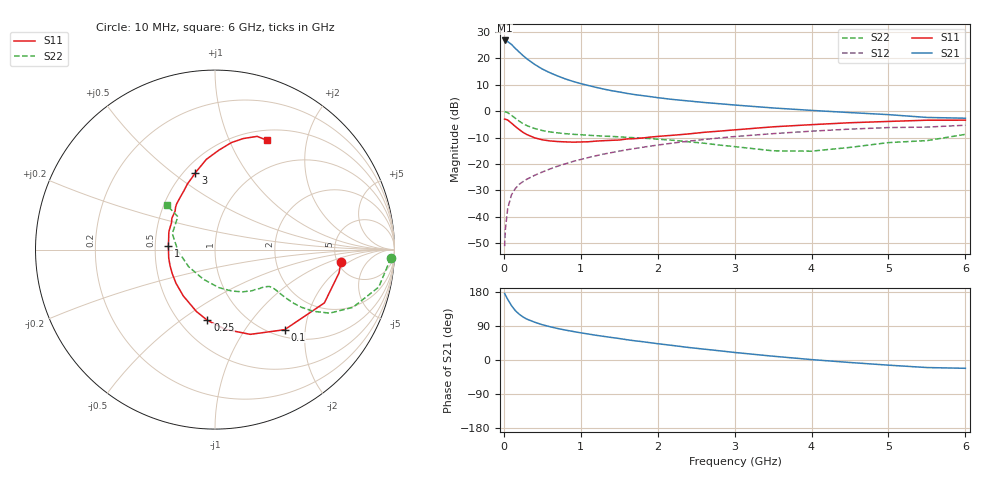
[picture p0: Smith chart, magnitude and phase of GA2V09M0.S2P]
! Infineon Technologies  Discrete & RF Semiconductors
! BF775
! Si NPN RF Bipolar Junction Transistor in SOT23
! VCE = 2 V  IC = 9 mA
! Common Emitter S-Parameters:  May  1996
# GHz  S  MA  R  50
!  f  S11  S21  S12  S22
! GHz  MAG  ANG  MAG  ANG  MAG  ANG  MAG  ANG
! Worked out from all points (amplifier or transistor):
!   36 points, 10 MHz to 6 GHz, reference 50 ohm
!   highest |S21| = 26.7 dB at 10 MHz (marker M1)
!   |S21| within 3 dB of that: start of sweep to 149.3 MHz
!   unconditionally stable (mu >= 1): 562.9 MHz to 3.79 GHz
!   at 250 MHz: K = 0.67, MSG = 23.8 dB, |S12| = -26.6 dB
!   at 1.4 GHz: K = 1.13, MAG = 9.5 dB, |S12| = -15.7 dB
!   at 6 GHz: K = 0.98, MSG = 1.3 dB, |S12| = -5.3 dB
!   S11 on the Smith chart (normalised r, x): 10 MHz: 5.39, -1.45; 100 MHz: 1.13, -1.56; 250 MHz: 0.68, -0.63; 1 GHz: 0.59, +0.03; 3 GHz: 0.57, +0.60; 6 GHz: 0.62, +1.39
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0.01  0.7057 -5.5  21.65 175.8  0.0028 87.3  0.9808 -2.7
0.02  0.703 -10.7  21.42 171.5  0.0058 85.7  0.9666 -5.3
0.05  0.6779 -26.0  20.59 160.1  0.0144 76.9  0.9358 -12.9
0.1  0.5913 -49.0  18.18 143.4  0.0263 69.4  0.8332 -22.7
0.15  0.5115 -67.4  15.29 130.1  0.0345 63.4  0.7302 -29.0
0.2  0.4482 -82.6  13.07 120.8  0.0413 60.9  0.647 -32.1
0.25  0.3961 -96.2  11.18 113.4  0.0466 59.5  0.5788 -33.7
0.3  0.3601 -106.7  9.709 107.8  0.0517 59.8  0.5313 -34.3
0.4  0.3128 -124.4  7.653 99.8  0.0611 59.6  0.4694 -34.3
0.5  0.2869 -139.3  6.242 93.1  0.0706 61.1  0.4294 -33.9
0.6  0.2732 -150.8  5.306 87.8  0.0806 61.8  0.4042 -33.5
0.7  0.266 -160.3  4.612 83.1  0.0911 62.3  0.3877 -33.5
0.8  0.262 -169.9  4.058 79.0  0.1009 62.2  0.3745 -33.8
1  0.261 175.0  3.311 71.7  0.1218 62.1  0.3577 -35.1
1.1  0.2634 168.7  3.043 68.5  0.1327 61.7  0.3497 -36.4
1.6  0.2973 143.9  2.163 53.5  0.1861 58.2  0.3193 -43.8
2.2  0.3499 123.7  1.658 38.2  0.2493 52.0  0.2812 -56.9
3  0.4417 104.4  1.304 19.9  0.3304 42.2  0.2133 -84.0
3.5  0.5049 95.5  1.147 10.0  0.3753 35.4  0.1774 -111.7
4.5  0.603 81.3  0.938 -6.6  0.4569 22.0  0.206 -177.8
5.5  0.6731 69.6  0.759 -19.9  0.4988 7.6  0.277 138.4
6  0.6741 64.8  0.734 -21.9  0.5408 3.6  0.3633 137.3
